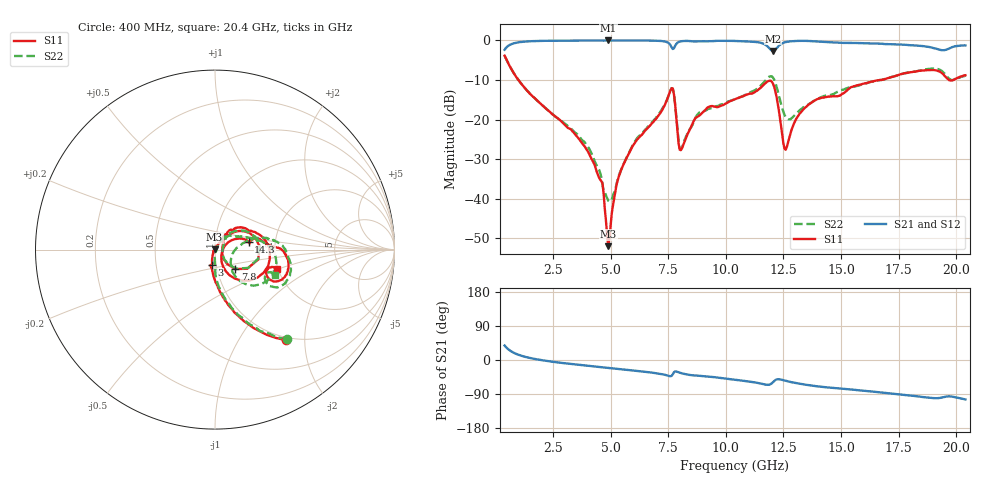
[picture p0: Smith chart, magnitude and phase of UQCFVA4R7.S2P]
!  Part Number  UQCFVA4R7  Mounting Orientation: Horizontal
!  Description: Ultra Low ESR Microwave capacitors
!  Application: Coupling, Bypass, Tuning, DC Block
!  Filters, Matching
# GHZ S DB R 50
! Freq  |S11|  S11 Ph  |S21|  S21 Ph  |S12|  S12 Ph  |S22|  S22 Ph
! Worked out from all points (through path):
!   401 points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, 400 MHz to 20.4 GHz, reference 50 ohm
!   highest |S21| = 0.00 dB at 4.9 GHz (marker M1); lowest = -2.7 dB at 12.05 GHz (marker M2)
!   group delay of S21, straight-line fit = 16 ps
!   lowest |S11| = -52.0 dB at 4.9 GHz (marker M3), VSWR 1.01, Z = 49.8 + j0.109 ohm
!   |S11| at or under -10 dB: 998.8 MHz to 16.69 GHz (15.69 GHz wide, 177 % of centre); 19.69 GHz to 19.89 GHz (199.2 MHz wide, 1.01 % of centre)
!   |S22| runs from -40.8 to -3.9 dB; largest |S21 - S12| = 0.0078
!   S11 on the Smith chart (normalised r, x): 400 MHz: 0.95, -1.63; 3 GHz: 0.95, -0.16; 7.8 GHz: 1.22, -0.27; 14.3 GHz: 1.45, +0.13; 20.4 GHz: 1.98, -0.50
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0.4  -3.85 -51.9  -2.35 38.2  -2.35 38.0  -3.86 -51.2
1.15  -11.15 -79.5  -0.35 10.8  -0.36 10.8  -11.10 -78.5
3  -21.25 -101.3  -0.07 -8.5  -0.07 -8.6  -20.98 -89.5
3.75  -25.85 -107.5  -0.03 -13.6  -0.03 -13.7  -25.10 -91.3
4.6  -35.60 -119.2  -0.02 -19.1  -0.03 -19.1  -34.61 -83.5
4.9  -52.03 154.0  0.00 -20.8  0.00 -20.9  -40.53 -32.0
5.55  -31.49 60.6  -0.01 -24.9  -0.01 -25.1  -31.36 50.9
7.1  -18.83 46.0  -0.09 -36.0  -0.10 -36.0  -18.55 49.3
7.6  -12.58 16.3  -1.19 -42.9  -1.20 -42.9  -12.59 17.9
7.8  -16.13 -44.0  -1.36 -30.1  -1.36 -30.2  -16.03 -42.0
8.05  -27.75 3.3  -0.23 -34.4  -0.22 -34.3  -27.59 -1.2
8.85  -19.02 53.4  -0.22 -41.8  -0.21 -41.6  -18.25 40.0
10.4  -14.90 43.0  -0.13 -52.2  -0.12 -52.0  -14.88 22.7
11.55  -11.78 19.6  -0.65 -62.6  -0.65 -62.6  -11.24 8.2
12.05  -10.94 -33.2  -2.68 -58.4  -2.67 -58.3  -9.39 -30.9
12.6  -27.65 -12.1  -0.41 -55.0  -0.40 -55.1  -19.40 -34.7
13.1  -19.44 29.5  -0.12 -61.5  -0.11 -61.5  -18.22 4.8
13.75  -15.60 20.9  -0.19 -67.6  -0.17 -67.7  -15.55 13.6
14.3  -14.33 12.6  -0.39 -71.7  -0.39 -71.4  -14.05 13.5
17.1  -9.42 2.4  -0.94 -88.0  -0.95 -88.0  -9.41 8.2
19.4  -8.35 -27.6  -2.47 -98.8  -2.46 -98.9  -7.82 -31.2
20.4  -8.79 -17.5  -1.25 -104.0  -1.23 -104.0  -8.85 -22.7
